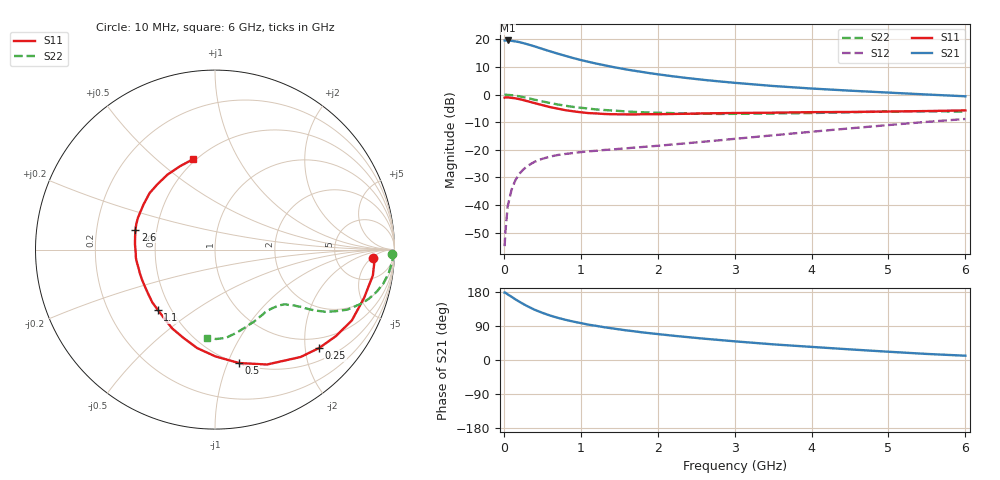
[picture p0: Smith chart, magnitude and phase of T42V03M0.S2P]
! Infineon Technologies  Discrete & RF Semiconductors
! BFR182T
! Si NPN RF Bipolar Junction Transistor in SC75
! VCE = 2 V  IC = 3 mA
! Common Emitter S-Parameters:  October  1999
# GHz  S  MA  R  50
!  f  S11  S21  S12  S22
! GHz  MAG  ANG  MAG  ANG  MAG  ANG  MAG  ANG
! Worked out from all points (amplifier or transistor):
!   36 points, 10 MHz to 6 GHz, reference 50 ohm
!   highest |S21| = 19.6 dB at 50 MHz (marker M1)
!   |S21| within 3 dB of that: start of sweep to 495.2 MHz
!   unconditionally stable (mu >= 1): 1.684 GHz to 4.217 GHz
!   at 250 MHz: K = 0.20, MSG = 23.0 dB, |S12| = -27.2 dB
!   at 1.4 GHz: K = 0.90, MSG = 15.0 dB, |S12| = -19.9 dB
!   at 6 GHz: K = 0.84, MSG = 4.1 dB, |S12| = -8.8 dB
!   lowest NFmin = 1.10 dB at 450 MHz
!   S11 on the Smith chart (normalised r, x): 10 MHz: 14, -6; 250 MHz: 0.76, -2.30; 500 MHz: 0.51, -1.10; 1.1 GHz: 0.42, -0.36; 2.6 GHz: 0.38, +0.11; 6 GHz: 0.48, +0.67
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0.01  0.882 -2.9  9.552 178.0  0.0018 86.7  0.9878 -1.5
0.02  0.8923 -2.4  9.56 177.6  0.0032 90.1  0.9988 -1.6
0.05  0.8912 -9.3  9.577 173.2  0.0095 86.5  0.9891 -3.9
0.1  0.8732 -17.9  9.42 166.9  0.0189 81.7  0.9769 -7.7
0.15  0.8586 -27.3  9.212 160.1  0.0282 75.2  0.9569 -11.3
0.2  0.8287 -35.5  8.945 154.0  0.0367 72.8  0.932 -14.5
0.25  0.7985 -43.3  8.587 148.2  0.0435 67.5  0.9021 -17.5
0.3  0.7654 -51.4  8.217 142.6  0.0504 64.4  0.8734 -20.0
0.4  0.7026 -65.7  7.485 132.6  0.0608 58.4  0.8098 -24.4
0.5  0.6457 -78.1  6.746 124.6  0.0688 54.1  0.754 -27.1
0.6  0.595 -89.8  6.092 117.4  0.0754 50.7  0.7059 -29.4
0.8  0.5227 -109.6  5.042 106.1  0.0842 47.3  0.6296 -32.1
0.9  0.4997 -118.5  4.606 101.5  0.0876 46.4  0.6001 -33.0
1.1  0.4631 -133.4  3.932 93.3  0.094 45.3  0.5581 -34.5
1.3  0.4467 -146.3  3.425 86.7  0.0993 45.9  0.5272 -36.0
1.6  0.4391 -162.2  2.845 78.0  0.1068 47.2  0.495 -38.0
2.2  0.4466 176.5  2.146 64.1  0.1253 51.8  0.462 -44.0
2.6  0.457 165.9  1.849 56.3  0.1406 54.4  0.4502 -48.9
3.5  0.4709 147.7  1.434 41.3  0.1833 58.3  0.4554 -60.9
4.5  0.4853 131.3  1.18 28.0  0.245 58.3  0.4785 -75.4
5.5  0.5042 112.5  1.005 16.0  0.3211 54.8  0.4981 -89.2
6  0.5182 103.6  0.933 11.3  0.3625 51.6  0.4947 -95.3
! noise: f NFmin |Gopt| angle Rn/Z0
0.45  1.1  0.37  30  0.33
0.9  1.2  0.35  61  0.26
1.8  1.85  0.27  133  0.2
